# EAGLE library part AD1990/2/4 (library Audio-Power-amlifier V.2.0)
Manufactured after 2006. The AD199x is a two channel Bridge Tied Load (BTL) switching audio power amplifier with integrated ΣΔ modulator. The modulator accepts a 1Vrms input signal (maximum power) and generates a switching waveform to drive speakers directly. One of the two modulators can control both output stages providing twice the current for single-channel applications. A digital, microcontroller-compatible interface provides control of reset, mute and PGA gain as well as output signals for thermal and over-current error conditions. The output stage can operate from supply voltages ranging from 8V to 20V. The analog modulator and digital logic operate from a 5V supply.
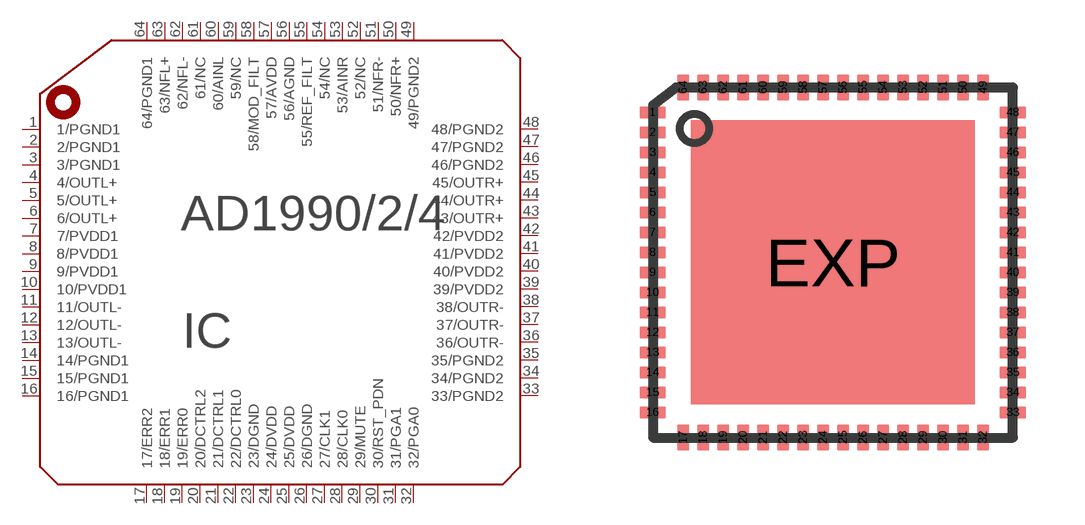
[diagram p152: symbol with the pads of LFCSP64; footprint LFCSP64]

Designator prefix IC

## AD1990/2/4  [LFCSP64]
1  1/PGND1  pwr
2  2/PGND1  pwr
3  3/PGND1  pwr
4  4/OUTL+  out
5  5/OUTL+  out
6  6/OUTL+  out
7  7/PVDD1  pwr
8  8/PVDD1  pwr
9  9/PVDD1  pwr
10  10/PVDD1  pwr
11  11/OUTL-  out
12  12/OUTL-  out
13  13/OUTL-  out
14  14/PGND1  pwr
15  15/PGND1  pwr
16  16/PGND1  pwr
17  17/ERR2  out
18  18/ERR1  out
19  19/ERR0  out
20  20/DCTRL2  in
21  21/DCTRL1  in
22  22/DCTRL0  in
23  23/DGND  pwr
24  24/DVDD  pwr
25  25/DVDD  pwr
26  26/DGND  pwr
27  27/CLK1  in
28  28/CLK0  out
29  29/MUTE  in
30  30/RST_PDN  in
31  31/PGA1  in
32  32/PGA0  in
33  33/PGND2  pwr
34  34/PGND2  pwr
35  35/PGND2  pwr
36  36/OUTR-  out
37  37/OUTR-  out
38  38/OUTR-  out
39  39/PVDD2  pwr
40  40/PVDD2  pwr
41  41/PVDD2  pwr
42  42/PVDD2  pwr
43  43/OUTR+  out
44  44/OUTR+  out
45  45/OUTR+  out
46  46/PGND2  pwr
47  47/PGND2  pwr
48  48/PGND2  pwr
49  49/PGND2  pwr
50  50/NFR+  in
51  51/NFR-  in
52  52/NC  nc
53  53/AINR  in
54  54/NC  nc
55  55/REF_FILT  out
56  56/AGND  pwr
57  57/AVDD  pwr
58  58/MOD_FILT  out
59  59/NC  nc
60  60/AINL  out
61  61/NC  nc
62  62/NFL-  in
63  63/NFL+  in
64  64/PGND1  pwr

## Footprint LFCSP64 (pad centres in mm)
64-Lead Lead Frame Chip Scale Package [LFCSP] CP-64-3 9 x 8,75 mm Body Source: http://www.analog.com/UploadedFiles/Packages/40887351787287CP_64_3.pdf
smd 0.65 x 0.3: 1 -4.515,3.75; 2 -4.515,3.25; 3 -4.515,2.75; 4 -4.515,2.25; 5 -4.515,1.75; 6 -4.515,1.25; 7 -4.515,0.75; 8 -4.515,0.25; 9 -4.515,-0.25; 10 -4.515,-0.75; 11 -4.515,-1.25; 12 -4.515,-1.75; 13 -4.515,-2.25; 14 -4.515,-2.75; 15 -4.515,-3.25; 16 -4.515,-3.75; 33 4.495,-3.75; 34 4.495,-3.25; 35 4.495,-2.75; 36 4.495,-2.25; 37 4.495,-1.75; 38 4.495,-1.25; 39 4.495,-0.75; 40 4.495,-0.25; 41 4.495,0.25; 42 4.495,0.75; 43 4.495,1.25; 44 4.495,1.75; 45 4.495,2.25; 46 4.495,2.75; 47 4.495,3.25; 48 4.495,3.75
smd 0.3 x 0.65: 17 -3.75,-4.375; 18 -3.25,-4.375; 19 -2.75,-4.375; 20 -2.25,-4.375; 21 -1.75,-4.375; 22 -1.25,-4.375; 23 -0.75,-4.375; 24 -0.25,-4.375; 25 0.25,-4.375; 26 0.75,-4.375; 27 1.25,-4.375; 28 1.75,-4.375; 29 2.25,-4.375; 30 2.75,-4.375; 31 3.25,-4.375; 32 3.75,-4.375; 49 3.75,4.375; 50 3.25,4.375; 51 2.75,4.375; 52 2.25,4.375; 53 1.75,4.375; 54 1.25,4.375; 55 0.75,4.375; 56 0.25,4.375; 57 -0.25,4.375; 58 -0.75,4.375; 59 -1.25,4.375; 60 -1.75,4.375; 61 -2.25,4.375; 62 -2.75,4.375; 63 -3.25,4.375; 64 -3.75,4.375
smd 7.1 x 7.1: EXP 0,0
